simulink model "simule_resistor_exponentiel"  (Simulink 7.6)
settings: Solver=ode15s  StartTime=0.0  StopTime=1  RelTol=1e-3
InitFcn:
  | R=5;
StartFcn:
  | clc
StopFcn:
  | close all
  | load  I_R_Simscape.mat
  | plotyy(x(1,:),x(2,:),x(1,:),x(3,:))
  | grid
  | title('Courant dans R et tension à ses bornes')
  | xlabel('Simulation d''une résistance non linéaire')
libraries: fl_lib x11, nesl_utility x6

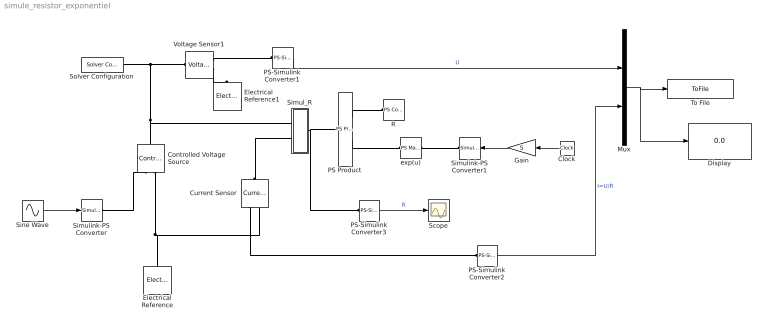
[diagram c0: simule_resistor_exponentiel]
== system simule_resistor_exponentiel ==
  Clock : Clock
  Controlled Voltage Source : fl_lib/Electrical/Electrical Sources/Controlled Voltage Source  DialogController=NetworkEngine.DynNeDlgSource  SystemSampleTime=-1  i_Log=off  v_Log=off  LocalVarNames=|i|v  LocalVarDescs=|i|v  LocalVarLogging=[0 0]
  Current Sensor : fl_lib/Electrical/Electrical Sensors/Current Sensor  DialogController=NetworkEngine.DynNeDlgSource  SystemSampleTime=-1  i1_Log=off  v1_Log=off  LocalVarNames=|i1|v1  LocalVarDescs=|i1|v1  LocalVarLogging=[0 0]
  Display : Display
  Electrical Reference : fl_lib/Electrical/Electrical Elements/Electrical Reference  DialogController=NetworkEngine.DynNeDlgSource  SystemSampleTime=-1  i_Log=off  LocalVarNames=|i  LocalVarDescs=|i  LocalVarLogging=0
  Electrical Reference1 : fl_lib/Electrical/Electrical Elements/Electrical Reference  DialogController=NetworkEngine.DynNeDlgSource  SystemSampleTime=-1  i_Log=off  LocalVarNames=|i  LocalVarDescs=|i  LocalVarLogging=0
  Gain : Gain  Gain=5
  Mux : Mux  Inputs=2
  PS Product : fl_lib/Physical Signals/Functions/PS Product  DialogController=NetworkEngine.DynNeDlgSource  SystemSampleTime=-1  LocalVarLogging=[]
  PS-Simulink Converter1 : nesl_utility/PS-Simulink Converter  DialogController=NetworkEngine.DynNeUtilDlgSource  SystemSampleTime=-1  PhysicalDomain=network_engine_domain  LeftPortType=input  RightPortType=output  SubClassName=ps_output  Unit=1  AffineConversion=off
  PS-Simulink Converter2 : nesl_utility/PS-Simulink Converter  DialogController=NetworkEngine.DynNeUtilDlgSource  SystemSampleTime=-1  PhysicalDomain=network_engine_domain  LeftPortType=input  RightPortType=output  SubClassName=ps_output  Unit=1  AffineConversion=off
  PS-Simulink Converter3 : nesl_utility/PS-Simulink Converter  DialogController=NetworkEngine.DynNeUtilDlgSource  SystemSampleTime=-1  PhysicalDomain=network_engine_domain  LeftPortType=input  RightPortType=output  SubClassName=ps_output  Unit=1  AffineConversion=off
  R : fl_lib/Physical Signals/Sources/PS Constant  DialogController=NetworkEngine.DynNeDlgSource  SystemSampleTime=-1  constant=R  LocalVarLogging=[]
  Scope : Scope
  Simul_R : Subsystem
  Simulink-PS Converter : nesl_utility/Simulink-PS Converter  DialogController=NetworkEngine.DynNeUtilDlgSource  SystemSampleTime=-1  PhysicalDomain=network_engine_domain  LeftPortType=input  RightPortType=output  SubClassName=ps_input  Unit=1  AffineConversion=off  InputFilterTimeConstant=.001  UdotUserProvided=0
  Simulink-PS Converter1 : nesl_utility/Simulink-PS Converter  DialogController=NetworkEngine.DynNeUtilDlgSource  SystemSampleTime=-1  PhysicalDomain=network_engine_domain  LeftPortType=input  RightPortType=output  SubClassName=ps_input  Unit=1  AffineConversion=off  InputFilterTimeConstant=.001  UdotUserProvided=0
  Sine Wave : Sin  Frequency=30  SampleTime=0
  Solver Configuration : nesl_utility/Solver Configuration  DialogController=NetworkEngine.DynNeUtilDlgSource  SystemSampleTime=-1  PhysicalDomain=network_engine_domain  LeftPortType=input  RightPortType=generic  SubClassName=solver  Accelerate=off  Profile=off  ResidualTolerance=1e-9  MaxNonlinIter=3  MaxModeIter=2  DoFixedCost=off  UseLocalSampling=off  DoDC=off  LinearAlgebra=Sparse  LocalSolverSampleTime=.001  LocalSolverChoice=NE_BACKWARD_EULER_ADVANCER  UseLocalSolver=off
  To File : ToFile  Filename=I_R_Simscape  MatrixName=x
  Voltage Sensor1 : fl_lib/Electrical/Electrical Sensors/Voltage Sensor  DialogController=NetworkEngine.DynNeDlgSource  SystemSampleTime=-1  i1_Log=off  v1_Log=off  LocalVarNames=|i1|v1  LocalVarDescs=|i1|v1  LocalVarLogging=[0 0]
  exp(u) : fl_lib/Physical Signals/Functions/PS Math Function  DialogController=NetworkEngine.DynNeDlgSource  SystemSampleTime=-1  fcn_choice=3  LocalVarLogging=[]
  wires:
  Sine Wave/1 -> Simulink-PS Converter/1
  PS-Simulink Converter1/1 -> Mux/1  "U"
  PS-Simulink Converter2/1 -> Mux/2  "I=U/R"
  Mux/1 -> To File/1, Display/1
  Gain/1 -> Simulink-PS Converter1/1
  Clock/1 -> Gain/1
  PS-Simulink Converter3/1 -> Scope/1  "R"
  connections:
  Controlled Voltage Source/RConn2 -- Electrical Reference/LConn1 -- Current Sensor/RConn2
  Simulink-PS Converter/RConn1 -- Controlled Voltage Source/RConn1
  Controlled Voltage Source/LConn1 -- Simul_R/LConn1 -- Voltage Sensor1/LConn1 -- Solver Configuration/RConn1
  Voltage Sensor1/RConn1 -- PS-Simulink Converter1/LConn1
  Voltage Sensor1/RConn2 -- Electrical Reference1/LConn1
  Current Sensor/LConn1 -- Simul_R/LConn2
  Current Sensor/RConn1 -- PS-Simulink Converter2/LConn1
  exp(u)/LConn1 -- Simulink-PS Converter1/RConn1
  PS Product/LConn1 -- R/RConn1
  PS Product/LConn2 -- exp(u)/RConn1
  Simul_R/RConn1 -- PS Product/RConn1 -- PS-Simulink Converter3/LConn1

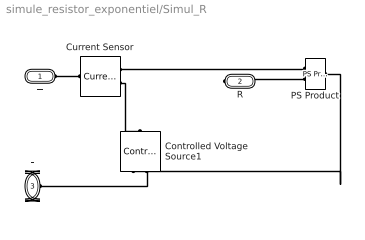
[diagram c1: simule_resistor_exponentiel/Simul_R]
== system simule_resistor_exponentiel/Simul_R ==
  Controlled Voltage Source1 : fl_lib/Electrical/Electrical Sources/Controlled Voltage Source  DialogController=NetworkEngine.DynNeDlgSource  SystemSampleTime=-1  i_Log=off  v_Log=off  LocalVarNames=|i|v  LocalVarDescs=|i|v  LocalVarLogging=[0 0]
  Current Sensor : fl_lib/Electrical/Electrical Sensors/Current Sensor  DialogController=NetworkEngine.DynNeDlgSource  SystemSampleTime=-1  i1_Log=off  v1_Log=off  LocalVarNames=|i1|v1  LocalVarDescs=|i1|v1  LocalVarLogging=[0 0]
  PS Product : fl_lib/Physical Signals/Functions/PS Product  DialogController=NetworkEngine.DynNeDlgSource  SystemSampleTime=-1  LocalVarLogging=[]
  + : PMIOPort  Port=1  Side=Left
  R : PMIOPort  Port=2  Side=Right
  - : PMIOPort  Port=3  Side=Left
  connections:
  Current Sensor/RConn2 -- Controlled Voltage Source1/LConn1
  PS Product/RConn1 -- Controlled Voltage Source1/RConn1
  Current Sensor/RConn1 -- PS Product/LConn1
  +/RConn1 -- Current Sensor/LConn1
  R/RConn1 -- PS Product/LConn2
  Controlled Voltage Source1/RConn2 -- -/RConn1
